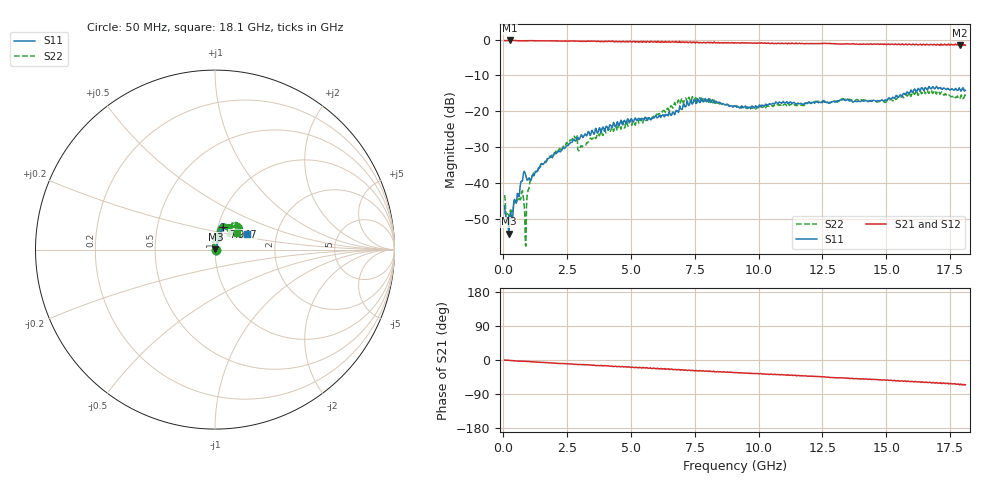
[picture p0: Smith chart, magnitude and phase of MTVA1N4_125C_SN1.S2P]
! Network Analyzer HP8720D.06.14 Serial No. US36140669
! 12 Jan 2005  09:08:50
! Frequency  S11  S21  S12  S22
# HZ  S  DB R 50
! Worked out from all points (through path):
!   801 points, 50 MHz to 18.1 GHz, reference 50 ohm
!   highest |S21| = -0.26 dB at 253.1 MHz (marker M1); lowest = -1.6 dB at 17.9 GHz (marker M2)
!   group delay of S21, straight-line fit = 9.67 ps
!   lowest |S11| = -54.1 dB at 207.9 MHz (marker M3), VSWR 1.00, Z = 50.2 + j0.0596 ohm
!   |S11| at or under -10 dB: start of sweep to end of sweep
!   |S22| runs from -57.6 to -14.1 dB; largest |S21 - S12| = 0.032
!   S11 on the Smith chart (normalised r, x): 50 MHz: 1.01, -0.00; 7.947 GHz: 1.06, +0.28; 18.1 GHz: 1.40, +0.25
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5e7  -46.27 -11.2  -0.29 -0.3  -0.29 -0.6  -43.34 1.1
2.079375e8  -54.08 17.5  -0.29 -0.8  -0.28 -1.1  -48.55 5.3
2.530625e8  -49.66 37.5  -0.26 -1.0  -0.27 -1.5  -48.15 13.1
6.8175e8  -39.82 72.6  -0.35 -3.0  -0.35 -3.4  -44.42 59.9
7.494375e8  -39.42 71.9  -0.35 -3.4  -0.35 -3.6  -42.13 48.6
7.945625e8  -37.09 68.9  -0.36 -3.4  -0.33 -3.6  -44.63 41.0
9.299375e8  -39.19 50.0  -0.32 -3.9  -0.33 -4.2  -43.74 119.1
9.97625e8  -38.60 55.3  -0.33 -4.3  -0.31 -4.6  -41.70 106.6
1.133e9  -37.82 71.6  -0.32 -4.9  -0.27 -5.3  -38.20 101.7
1.448875e9  -35.50 74.0  -0.39 -6.1  -0.37 -6.3  -34.98 101.8
2.802625e9  -28.17 65.0  -0.47 -11.4  -0.44 -11.8  -27.35 99.4
3.073375e9  -26.59 71.0  -0.47 -12.2  -0.45 -12.4  -29.69 94.6
4.043562e9  -24.16 64.3  -0.55 -15.6  -0.48 -15.3  -25.92 93.2
6.074188e9  -21.61 71.3  -0.61 -23.5  -0.61 -23.3  -20.86 81.7
7.066938e9  -17.86 72.3  -0.70 -27.2  -0.66 -26.6  -17.55 69.8
7.946875e9  -17.31 70.2  -0.90 -28.8  -0.78 -29.5  -16.82 54.0
9.075e9  -18.52 74.7  -0.94 -33.0  -0.88 -33.3  -18.61 45.0
1.209838e10  -17.69 61.8  -1.13 -42.8  -1.10 -43.2  -17.48 56.8
1.509919e10  -16.26 32.3  -1.30 -54.0  -1.19 -53.5  -17.10 58.1
1.652062e10  -13.39 27.9  -1.54 -59.1  -1.30 -59.0  -14.99 43.1
1.789694e10  -13.91 23.4  -1.63 -64.1  -1.66 -64.6  -16.35 42.0
1.81e10  -14.18 25.8  -1.57 -65.5  -1.57 -66.6  -16.12 36.7
